(* Logix 5000 AddOnInstructionDefinition export; software revision 16.00 *)

ADD_ON_INSTRUCTION AMCI_ANG1E_Immediate_Stop   (* revision 1.0, vendor AMCI *)
VAR_IN_OUT
   AMCI_ANG1E_output_data : INT[10]; {required}
END_VAR
VAR
   command_data_block : INT[10];
        [0]   // Command Bits MSW
        [1]   // Command Bits LSW
        [2]   // Upper Target Position
        [3]   // Lower Target Position
        [4]   // Upper Programmed Speed
        [5]   // Lower Programmed Speed
END_VAR

ROUTINE Logic   (* ladder *)
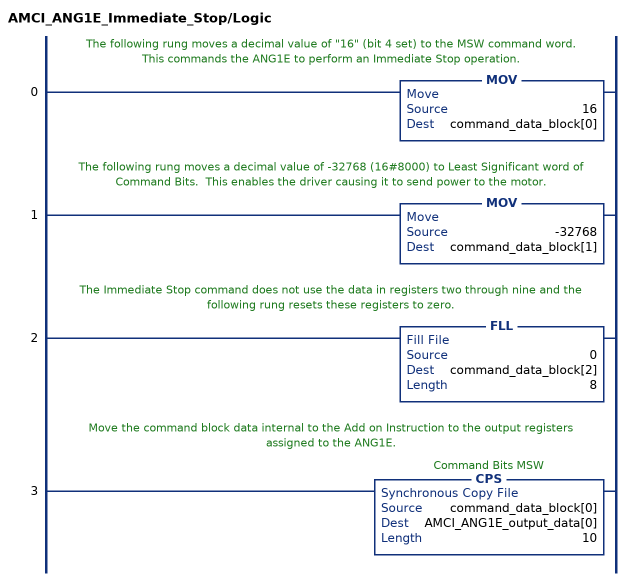
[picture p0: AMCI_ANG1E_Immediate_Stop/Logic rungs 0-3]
   // The following rung moves a decimal value of "16" (bit 4 set) to the MSW command word.  This commands the ANG1E to perform an Immediate Stop operation.
   0: MOV(16,command_data_block[0]);
   // The following rung moves a decimal value of -32768 (16#8000) to Least Significant word of Command Bits.  This enables the driver causing it to send power to the motor.
   1: MOV(-32768,command_data_block[1]);
   // The Immediate Stop command does not use the data in registers two through nine and the following rung resets these registers to zero.
   2: FLL(0,command_data_block[2],8);
   // Move the command block data internal to the Add on Instruction to the output registers assigned to the ANG1E.
   3: CPS(command_data_block[0],AMCI_ANG1E_output_data[0],10);
END_ROUTINE
END_ADD_ON_INSTRUCTION
